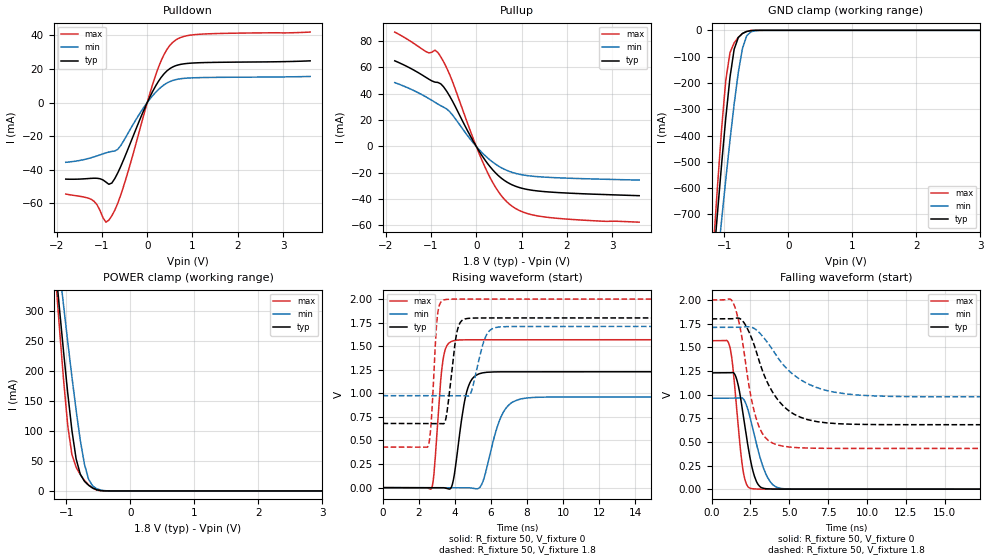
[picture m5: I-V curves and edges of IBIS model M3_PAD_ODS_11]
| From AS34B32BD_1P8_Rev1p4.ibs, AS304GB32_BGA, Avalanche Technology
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[Model] M3_PAD_ODS_11
Model_type I/O
Enable   Active-High
Vinl  =  0.63
Vinh  =  1.17
Vmeas =  0.9
Cref  =  30e-12
| Capacitance  typ   min   max
C_comp   6.492186e-12   6.071794e-12   6.967131e-12
| Variables   typ   min   max
[GND Clamp Reference]   0   0   0
[POWER Clamp Reference]   1.8   1.71   2
[Pulldown Reference]   0   0   0
[Pullup Reference]   1.8   1.71   2
[Temperature Range]   25   125   -40
[Voltage Range]   1.8   1.71   2
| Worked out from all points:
|   slope of the pulldown table from 0 to 0.27 V, typ, clamps not added: 20 ohm
|   slope of the pullup table from 0 to 0.27 V, typ, clamps not added: 19.4 ohm
|   GND clamp passes 1 mA (typ) near -0.58 V on its own axis
|   POWER clamp passes 1 mA (typ) near -0.48 V on its own axis
|   falling waveform, R_fixture 50, V_fixture 0: 20-80 % time 733ps typ, 955ps min, 536ps max; typ from 1.23 V to 0 V
|   falling waveform, R_fixture 50, V_fixture 1.8: 20-80 % time 1.84ns typ, 2.55ns min, 1.02ns max; typ from 1.8 V to 0.681 V
|   rising waveform, R_fixture 50, V_fixture 0: 20-80 % time 562ps typ, 856ps min, 364ps max; typ from 0 V to 1.23 V
|   rising waveform, R_fixture 50, V_fixture 1.8: 20-80 % time 410ps typ, 568ps min, 265ps max; typ from 0.681 V to 1.8 V
[GND Clamp]
| Voltage   I(typ)   I(min)   I(max)
-1.8V     -2.882A    -2.682A    -3.302A
-1.173V   -889.3mA   -1.041A    -830.7mA
-1.108V   -695.2mA   -879.1mA   -594mA
-1.043V   -507.9mA   -720.4mA   -373.2mA
-977.6mV  -332.2mA   -566.2mA   -188.7mA
-912.4mV  -178.9mA   -418.3mA   -84.9mA
-847.2mV  -71.94mA   -280.4mA   -47.66mA
-782.1mV  -27.06mA   -159.4mA   -26.61mA
-716.9mV  -11.75mA   -68.54mA   -12.18mA
-651.7mV  -4.473mA   -21mA      -3.801mA
-456.2mV  -15.91uA   -297.6uA   -1.681uA
3.6V      0A         0A         0A
[POWER Clamp]
| Voltage   I(typ)   I(min)   I(max)
-1.8V     1.148A     1.073A     1.318A
-1.173V   379.5mA    433.8mA    364.1mA
-1.108V   304.4mA    370.6mA    271.9mA
-1.043V   231.6mA    308.7mA    184.6mA
-977.6mV  162.5mA    248.2mA    108.6mA
-912.4mV  100.5mA    189.8mA    60.25mA
-847.2mV  53.5mA     134.6mA    39.41mA
-716.9mV  16.06mA    44.37mA    17.57mA
-651.7mV  9.361mA    19.28mA    9.931mA
-586.6mV  4.721mA    8.013mA    4.451mA
-325.9mV  4.613uA    79.39uA    440.6nA
3.6V      0A         0A         0A
[Pulldown]
| Voltage   I(typ)   I(min)   I(max)
-1.8V     -45.6mA    -35.58mA   -54.5mA
-1.238V   -45.15mA   -32.87mA   -57.63mA
-912.4mV  -47.36mA   -29.97mA   -71.26mA
-847.2mV  -48.69mA   -29.47mA   -70.02mA
-716.9mV  -45.3mA    -28.85mA   -64.14mA
-521.4mV  -34.03mA   -22.82mA   -49.79mA
-65.17mV  -3.915mA   -2.451mA   -6.278mA
248.3mV   12.65mA    7.772mA    20.97mA
434.5mV   18.83mA    11.62mA    31.58mA
620.7mV   21.87mA    13.59mA    37.09mA
1.179V    23.74mA    14.86mA    40.71mA
3.6V      24.84mA    15.54mA    41.96mA
[Pullup]
| Voltage   I(typ)   I(min)   I(max)
-1.8V     65.06mA    48.5mA     86.9mA
-1.108V   52.41mA    37.58mA    72.02mA
-912.4mV  48.87mA    33.57mA    73.19mA
-782.1mV  47.53mA    30.9mA     68.01mA
-521.4mV  34.19mA    23.72mA    48.98mA
-130.3mV  7.935mA    5.437mA    11.79mA
186.2mV   -9.992mA   -6.708mA   -15.2mA
496.6mV   -22.46mA   -15.07mA   -34.77mA
744.8mV   -28.41mA   -19.17mA   -44.22mA
1.055V    -32.21mA   -21.83mA   -50.2mA
1.49V     -34.31mA   -23.3mA    -53.53mA
3.6V      -37.46mA   -25.6mA    -57.6mA
[Ramp]
dV/dt_r   0.737574/0.562094n  0.576866/0.855605n  0.941388/0.363904n
dV/dt_f   0.67144/1.84014n  0.440568/2.55385n  0.941875/1.01591n
R_load = 50
[Falling Waveform]
R_fixture = 50
V_fixture = 0
V_fixture_min = 0
V_fixture_max = 0
| Time   V(typ)   V(min)   V(max)
0s        1.229V     961.4mV    1.569V
1.173ns   1.23V      961.8mV    1.506V
1.359ns   1.233V     961.8mV    1.308V
1.593ns   1.174V     961.9mV    892.5mV
1.986ns   839.4mV    962.2mV    239.8mV
2.457ns   346.3mV    770.9mV    10.98mV
3.061ns   35.62mV    368.2mV    1.068mV
3.613ns   3.252mV    120.1mV    699uV
4.376ns   832.3uV    10.37mV    190uV
21.88ns   78.27nV    103.8nV    1.429uV
[Falling Waveform]
R_fixture = 50
V_fixture = 1.8
V_fixture_min = 1.71
V_fixture_max = 2
| Time   V(typ)   V(min)   V(max)
0s        1.8V       1.71V      2V
1.427ns   1.804V     1.71V      1.957V
2.066ns   1.765V     1.715V     1.479V
2.432ns   1.653V     1.716V     1.067V
2.829ns   1.479V     1.689V     769.9mV
3.249ns   1.264V     1.623V     593mV
3.919ns   1.027V     1.475V     487.1mV
5.322ns   790.7mV    1.204V     441.1mV
8.081ns   692.7mV    1.02V      430.9mV
21.88ns   680.9mV    975.7mV    430.2mV
[Rising Waveform]
R_fixture = 50
V_fixture = 0
V_fixture_min = 0
V_fixture_max = 0
| Time   V(typ)   V(min)   V(max)
0s        3.56nV     168.5nV    2.623nV
2.714ns   -297.5uV   -531.5uV   -8.257mV
2.848ns   -312.2uV   -557.8uV   146.5mV
3.317ns   -363.5uV   -649.5uV   1.309V
3.797ns   -1.332mV   -743.6uV   1.549V
4.622ns   984.8mV    -905.3uV   1.568V
5.349ns   1.208V     -3.259mV   1.568V
6.542ns   1.228V     741.4mV    1.568V
7.449ns   1.228V     929mV      1.568V
21.88ns   1.229V     961.4mV    1.569V
[Rising Waveform]
R_fixture = 50
V_fixture = 1.8
V_fixture_min = 1.71
V_fixture_max = 2
| Time   V(typ)   V(min)   V(max)
0s        680.9mV    975.7mV    430.2mV
2.531ns   680.4mV    975.4mV    443.7mV
2.695ns   680.3mV    975.4mV    695.8mV
3.03ns    680.2mV    975.4mV    1.807V
3.387ns   677.9mV    975.3mV    1.99V
4.109ns   1.639V     975.3mV    2V
4.556ns   1.789V     975.2mV    2V
5.68ns    1.8V       1.587V     2V
6.217ns   1.8V       1.695V     2V
21.88ns   1.8V       1.71V      2V
